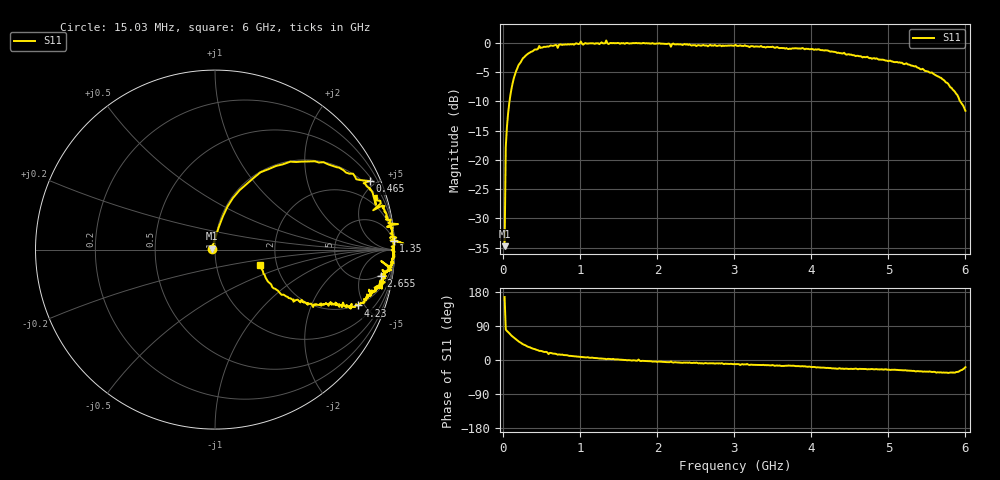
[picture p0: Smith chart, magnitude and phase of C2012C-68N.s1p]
!	Network	Analyzer	HP8753E.07.74:	Oct	30	2002	Serial	No.	JP38451487
!	Hewlett-Packard
!	7	Sep	2009	10:58:05
!	Frequency	S11
#	HZ	S	RI	R	50
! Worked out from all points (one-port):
!   400 points, 15.03 MHz to 6 GHz, reference 50 ohm
!   lowest |S11| = -34.7 dB at 15.03 MHz (marker M1), VSWR 1.04, Z = 48.2 + j0.425 ohm
!   |S11| at or under -10 dB: start of sweep to 78.67 MHz; 5.933 GHz to end of sweep
!   S11 on the Smith chart (normalised r, x): 15.03 MHz: 0.96, +0.01; 465 MHz: 0.68, +4.62; 1.35 GHz: 3, +39; 2.655 GHz: 4, -11; 4.23 GHz: 1.96, -4.47; 6 GHz: 1.63, -0.30
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1.502992e7  -0.0178 0.0044
3.002985e7  0.0217 0.127
6.00297e7  0.0693 0.239
9.002955e7  0.137 0.331
1.95029e8  0.42 0.49
4.650277e8  0.861 0.382
5.550272e8  0.863 0.341
5.850271e8  0.896 0.249
6.150269e8  0.902 0.305
7.650262e8  0.933 0.237
1.005025e9  1.02 0.142
1.035025e9  0.958 0.127
1.320023e9  0.994 0.056
1.335023e9  1.05 0.0331
1.350023e9  0.995 0.0502
1.515022e9  0.984 0.0165
1.755021e9  0.997 0.0206
2.145019e9  0.983 -0.0983
2.175019e9  0.926 -0.0638
2.265019e9  0.97 -0.109
2.655017e9  0.925 -0.148
3.015015e9  0.946 -0.183
3.765011e9  0.868 -0.232
4.230009e9  0.794 -0.311
4.515007e9  0.732 -0.314
5.265004e9  0.576 -0.308
5.685002e9  0.423 -0.272
6e9  0.249 -0.0851
